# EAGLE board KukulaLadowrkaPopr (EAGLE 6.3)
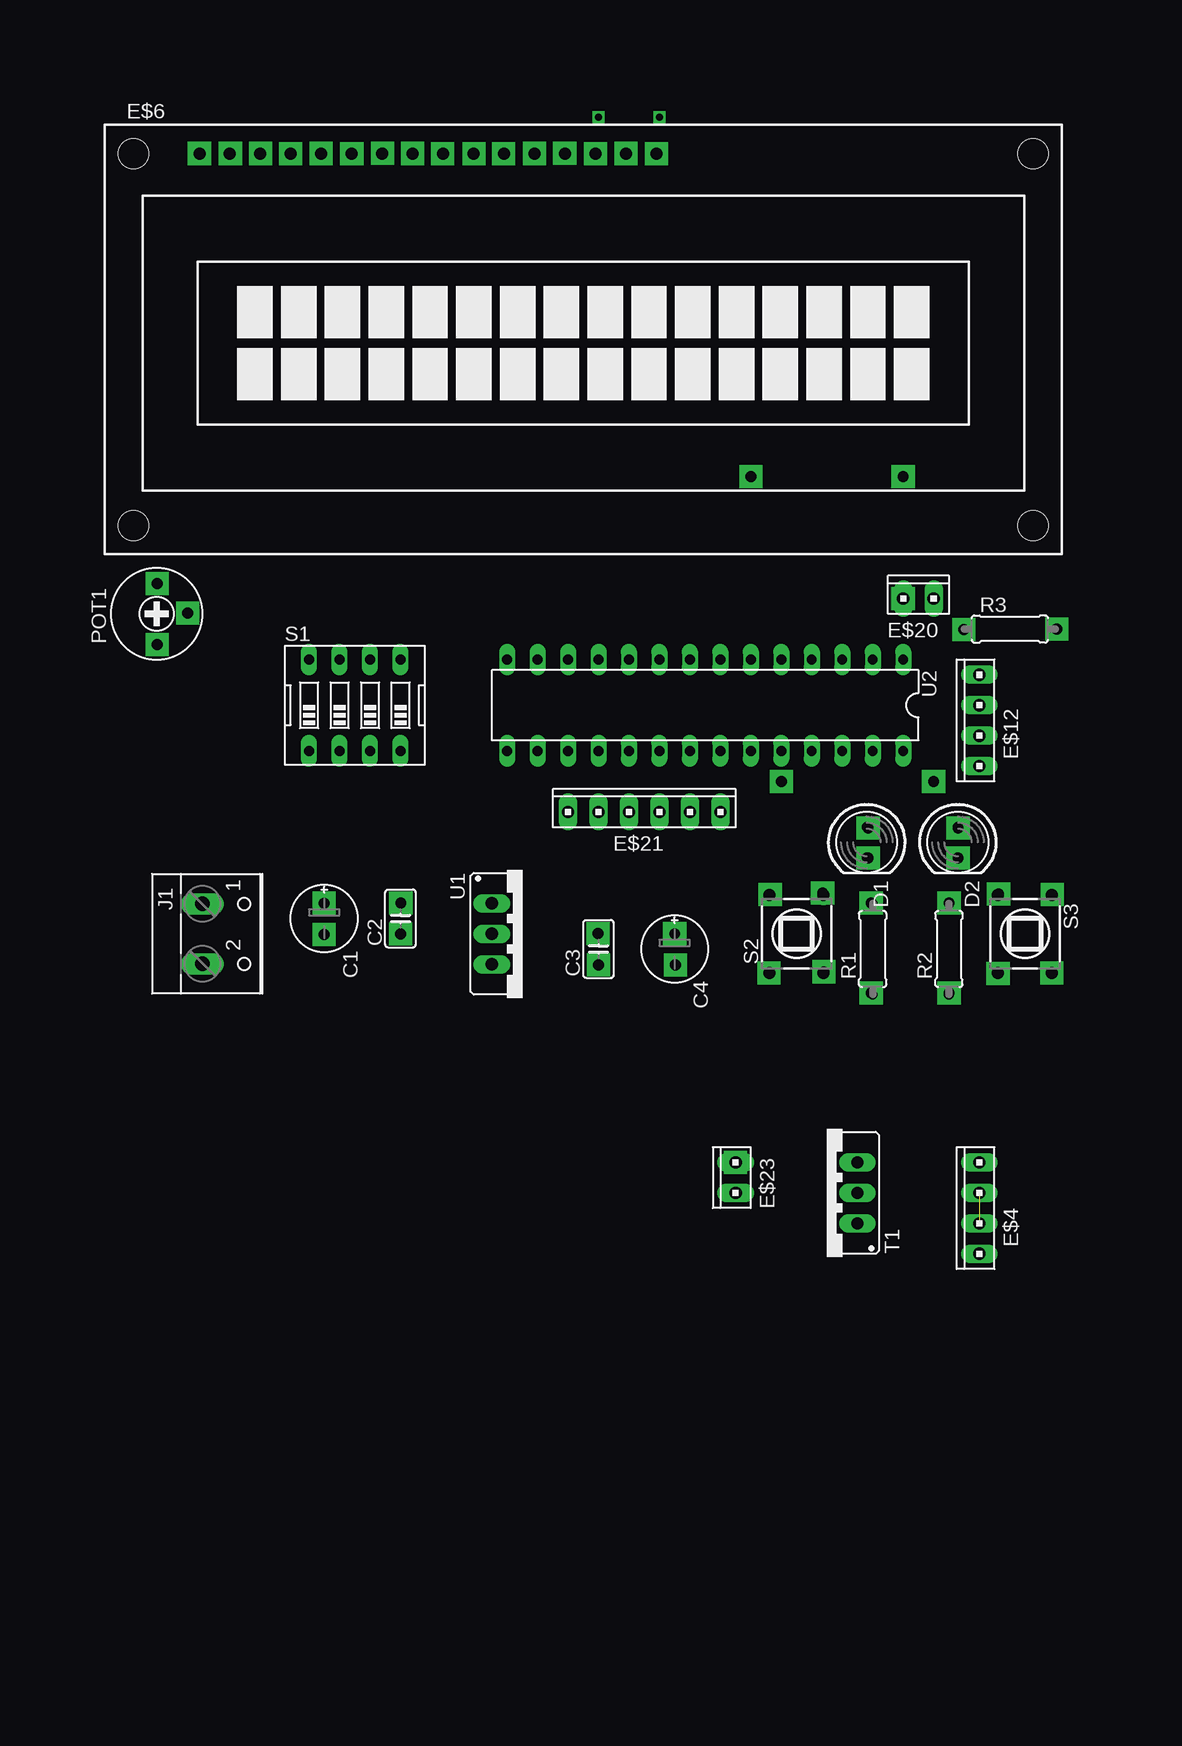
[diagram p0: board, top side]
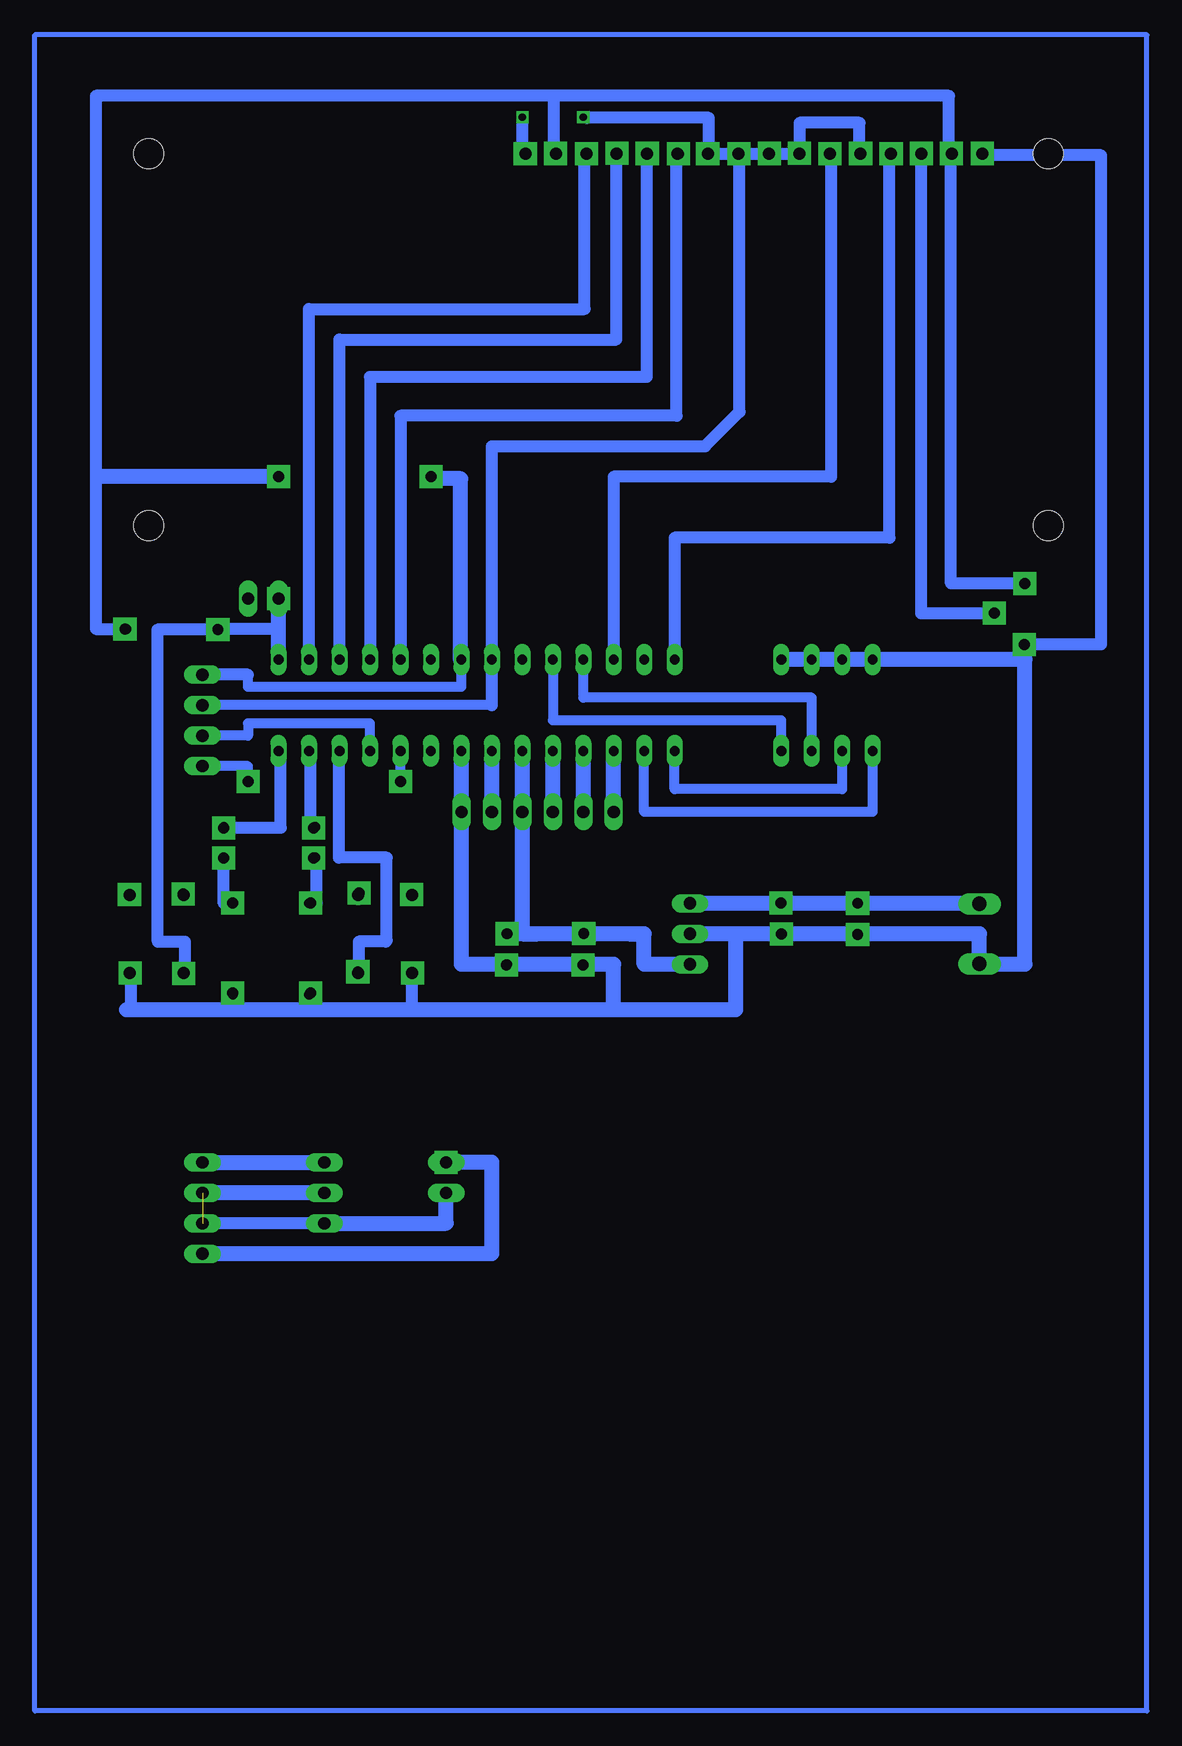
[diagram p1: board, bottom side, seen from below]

No outline drawn. Coordinates in mm, seen from the top.
Copper layers (1*16): Top 0.035mm / dielectric 1.5mm / Bottom 0.035mm
Design rules "default": minimum track width 10mil, minimum drill 24mil, track to track 8mil, track to pad 8mil, pad to pad 8mil, via to via 8mil, smd to smd 8mil, copper to edge 40mil, drill to drill 8mil, minimum pad ring 10mil, minimum via ring 8mil, stop-mask expansion 4mil, vias tented up to drill 0mil, thermal gap 10mil

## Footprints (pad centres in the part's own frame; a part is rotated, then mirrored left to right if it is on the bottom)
E2,5-6E = drill 0.813 pad 1.575: + -1.27,0 | drill 0.813 pad 1.575 octagon: - 1.27,0
C025-025X050 = drill 0.813 octagon: 1 -1.27,0; 2 1.27,0
LED5MM = drill 0.813 octagon: A -1.27,0; K 1.27,0
10X04MTA = drill 1.016 long: 1 3.81,0; 2 1.27,0; 3 -1.27,0; 4 -3.81,0
TUXGR_16X2_R2 = drill 1 pad 1.676: 1 -32,15.5; 2 -29.46,15.5; 3 -26.92,15.5; 4 -24.38,15.5; 5 -21.84,15.5; 6 -19.3,15.5; 7 -16.76,15.5; 8 -14.22,15.5; 9 -11.68,15.5; 10 -9.14,15.5; 11 -6.6,15.5; 12 -4.06,15.5; 13 -1.52,15.5; 14 1.02,15.5; 15 3.56,15.5; 16 6.1,15.5 | hole 2.5: -37.5,-15.5; 37.5,-15.5; -37.5,15.5; 37.5,15.5
10X02MTA = drill 1.016 long: 1 1.27,0; 2 -1.27,0
10X06MTA = drill 1.016 long: 1 6.35,0; 2 3.81,0; 3 1.27,0; 4 -1.27,0; 5 -3.81,0; 6 -6.35,0
W237-102 = drill 1.194 long: 1 -2.5,-1.27; 2 2.5,-1.27
RTRIM3339P = drill 0.61: 1 -2.54,0; 2 0,-2.54; 3 2.54,0
0207/7 = drill 0.813 octagon: 1 -3.81,0; 2 3.81,0
EDG-04 = drill 0.813 long: 1 -3.81,-3.81; 2 -1.27,-3.81; 3 1.27,-3.81; 4 3.81,-3.81; 5 3.81,3.81; 6 1.27,3.81; 7 -1.27,3.81; 8 -3.81,3.81
TL1105SP = drill 1 pad 1.676: 1 -2.25,3.25; 2 2.25,3.25; 3 -2.25,-3.25; 4 2.25,-3.25
78XXS = drill 1.016 long: GND 0,-2.54; IN -2.54,-2.54; OUT 2.54,-2.54
DIL28-3 = drill 0.813 long: 1 -16.51,-3.81; 2 -13.97,-3.81; 3 -11.43,-3.81; 4 -8.89,-3.81; 5 -6.35,-3.81; 6 -3.81,-3.81; 7 -1.27,-3.81; 8 1.27,-3.81; 9 3.81,-3.81; 10 6.35,-3.81; 11 8.89,-3.81; 12 11.43,-3.81; 13 13.97,-3.81; 14 16.51,-3.81; 15 16.51,3.81; 16 13.97,3.81; 17 11.43,3.81; 18 8.89,3.81; 19 6.35,3.81; 20 3.81,3.81; 21 1.27,3.81; 22 -1.27,3.81; 23 -3.81,3.81; 24 -6.35,3.81; 25 -8.89,3.81; 26 -11.43,3.81; 27 -13.97,3.81; 28 -16.51,3.81

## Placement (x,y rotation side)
C1  [E2,5-6E]  10.16,11.43 270 top
C2  [C025-025X050]  16.51,11.43 90 top
C3  [C025-025X050]  33.02,8.89 90 top
C4  [E2,5-6E]  39.37,8.89 270 top
D1  [LED5MM]  55.38,17.78 270 top
D2  [LED5MM]  62.98,17.78 270 top
E$4  [10X04MTA]  64.77,-12.7 90 top
E$6  U3  [TUXGR_16X2_R2]  31.75,59.69 0 top
E$12  [10X04MTA]  64.77,27.94 90 top
E$20  [10X02MTA]  59.69,38.1 0 top
E$21  [10X06MTA]  36.83,20.32 0 top
E$23  [10X02MTA]  44.45,-10.16 90 top
J1  [W237-102]  1.27,10.16 270 top
POT1  [RTRIM3339P]  -3.81,36.83 90 top
R1  [0207/7]  55.88,8.89 90 top
R2  [0207/7]  62.23,8.89 90 top
R3  [0207/7]  67.31,35.56 0 top
S1  [EDG-04]  12.7,29.21 0 top
S2  [TL1105SP]  49.53,10.16 0 top
S3  [TL1105SP]  68.58,10.16 180 top
T1  [78XXS]  52.07,-11.43 90 top
U1  [78XXS]  26.67,10.16 270 top
U2  [DIL28-3]  41.91,29.21 180 top

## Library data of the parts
C1-C4 POT1 R1-R3 = rcl
D1 D2 = led
E$4 E$12 E$20 E$21 E$23 = con-amp
E$6 = display-lcd
J1 = con-wago-500
S1 = special
S2 S3 = switch
T1 U1 = v-reg
U2 = fairchild-semic

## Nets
S$1: POT1.1 S1.5 U1.GND U2.22
S$2: U2.21
S$3: U1.OUT U2.20
S$4: U2.19
S$6: U2.17
S$7: R3.1 U2.1
S$8: U2.4
S$9: U2.5
S$10: U1.IN
S$11: S1.2 U2.15
S$12: S1.1 U2.16
S$13: U2.24
S$14: S1.4
S$15: S1.3
S$16: U2.2
S$17: U2.3
S$19: U2.12
S$21: U2.14
S$24: R3.2
S$26: U2.7
S$69: U2.8
S$72: R1.2
S$73: R2.2
S$87: U2.25
S$88: E$12.4
S$90: E$4.4
S$93: E$4.3 E$23.2 T1.IN
S$94: E$4.1 T1.OUT

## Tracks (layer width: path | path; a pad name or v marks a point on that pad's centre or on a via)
S$1
  Bottom 1.016: -0.24,75.04 -10.16,75.04 -10.16,34.29 POT1.1 -3.81,33.02
  Bottom 1.27: U2.22 43.18,7.62 30.48,7.62 30.48,3.81 27.94,3.81 | 27.94,3.81 20.32,3.81 20.32,10.16 | S1.5 -3.81,33.02 -3.81,7.62 0,7.62 0,10.16 20.32,10.16 | 20.32,10.16 U1.GND | 27.94,3.81 49.53,3.81 | 27.94,3.81 68.58,3.81 | 68.58,3.81 69.85,3.81 | 68.58,3.81 71.12,3.81
S$2
  Bottom 1.27: 40.64,20.32 U2.21
S$3
  Bottom 1.27: 29.21,10.16 28.57,10.16 | 29.21,10.16 38.1,10.16 | 38.1,10.16 36.83,10.16 | 38.1,10.16 U2.20 | U1.OUT 27.94,7.62 27.94,10.16 29.21,10.16
S$4
  Bottom 1.27: 35.56,20.32 U2.19
S$5
  Bottom 1.27: 33.02,20.32 33.02,25.4
S$6
  Bottom 1.27: 30.48,20.32 U2.17
S$7  (via drill 0.9 pad 1.93)
  Bottom 1.016: 58.42,35.56 R3.1
  Bottom 1.27: U2.1 58.42,35.56 v58.42,38.1
S$8
  Bottom 1.016: 27.72,75.13 27.72,56.56 50.8,56.56 U2.4
S$9
  Bottom 1.016: 25.25,75.13 25.25,53.34 48.26,53.34 U2.5
S$10
  Bottom 1.27: 0,12.7 U1.IN
S$11
  Bottom 0.813: U2.15 25.4,22.23 11.43,22.23 S1.2
S$12
  Bottom 0.813: U2.16 27.94,20.32 8.89,20.32 S1.1
S$13  (via drill 0.9 pad 1.93)
  Bottom 0.813: v48.26,22.86 U2.24
S$14
  Bottom 0.813: 35.56,27.94 16.51,27.94 S1.4
S$15
  Bottom 0.813: 33.02,29.84 13.97,29.84 S1.3
S$16
  Bottom 1.016: 32.9,75.21 32.9,62.23 55.88,62.23 U2.2
S$17
  Bottom 1.016: 30.27,75.04 30.27,59.69 53.34,59.69 U2.3
S$18
  Bottom 1.016: 22.61,75.21 22.61,75.16 14.96,75.16
S$19
  Bottom 1.016: 12.34,75.21 12.34,48.26 30.48,48.26 U2.12
S$20
  Bottom 1.016: 10,75.25 10,77.75 15,77.75 15,75.25
S$21
  Bottom 1.016: 7.48,75.21 7.48,43.18 25.4,43.18 U2.14
S$22
  Bottom 1.016: 4.85,75.29 4.85,36.86 -1.32,36.86
S$23
  Bottom 1.016: 2.37,75.04 2.37,39.36 -3.79,39.36
S$24  (via drill 0.9 pad 1.93)
  Bottom 1.016: 2.54,74.93 2.54,80.01 73.66,80.01 73.66,35.56 v71.23,35.56 R3.2
S$25  (via drill 0.9 pad 1.93)
  other vias: 45.72,48.26
S$26
  Bottom 0.813: U2.7 43.18,30.73 60.96,30.73 60.96,31.75
  Bottom 1.016: 60.96,31.75 64.77,31.75
S$27  (via drill 0.9 pad 1.93)
  Bottom 1.016: 55.75,25.25 55.75,18.98 v55.5,18.98
S$28  (via drill 0.9 pad 1.93)
  Bottom 1.27: v39.38,10.16 38,10.16 38,10.28
S$29  (via drill 0.9 pad 1.93)
  other vias: -3.76,34.27
S$30  (via drill 0.9 pad 1.93)
  other vias: -1.24,36.88
S$31  (via drill 0.9 pad 1.93)
  other vias: -3.78,39.34
S$32  (via drill 0.9 pad 1.93)
  other vias: 37.86,75.19
S$33  (via drill 0.9 pad 1.93)
  other vias: 35.32,75.21
S$34  (via drill 0.9 pad 1.93)
  other vias: 32.76,75.19
S$35  (via drill 0.9 pad 1.93)
  other vias: 30.21,75.23
S$36  (via drill 0.9 pad 1.93)
  other vias: 27.69,75.21
S$37  (via drill 0.9 pad 1.93)
  other vias: 25.09,75.17
S$38  (via drill 0.9 pad 1.93)
  other vias: 22.65,75.17
S$39  (via drill 0.9 pad 1.93)
  other vias: 20.03,75.19
S$40  (via drill 0.9 pad 1.93)
  other vias: 17.51,75.21
S$41  (via drill 0.9 pad 1.93)
  other vias: 15.01,75.23
S$42  (via drill 0.9 pad 1.93)
  other vias: 12.46,75.19
S$43  (via drill 0.9 pad 1.93)
  other vias: 9.9,75.21
S$44  (via drill 0.9 pad 1.93)
  other vias: 7.35,75.19
S$45  (via drill 0.9 pad 1.93)
  other vias: 4.84,75.21
S$46  (via drill 0.9 pad 1.93)
  other vias: 2.33,75.21
S$47  (via drill 0.9 pad 1.93)
  other vias: -0.25,75.21
S$48  (via drill 0.9 pad 1.93)
  other vias: 32.98,10.19
S$49  (via drill 0.9 pad 1.93)
  other vias: 33.03,7.55
S$50  (via drill 0.9 pad 1.93)
  other vias: 39.43,7.57
S$51  (via drill 0.9 pad 1.93)
  other vias: 16.54,12.73
S$52  (via drill 0.9 pad 1.93)
  other vias: 16.51,10.14
S$53  (via drill 0.9 pad 1.93)
  other vias: 10.15,12.71
S$54  (via drill 0.9 pad 1.93)
  other vias: 10.15,10.11
S$55
  Bottom 1.016: 70.7,6.79 70.71,3.8 47.29,3.8 | 47.29,3.8 47.28,6.85 | 47.28,3.81 47.29,3.8
S$56
  Bottom 1.016: 68.51,9.64 68.51,35.46
S$57  (via drill 0.9 pad 1.93)
  other vias: 63.48,35.51
S$58
  Bottom 1.016: 53.39,25.36 53.39,16.5 49.4,16.5 49.4,9.61
S$59  (via drill 0.9 pad 1.93)
  other vias: 47.33,13.42
S$60  (via drill 0.9 pad 1.93)
  other vias: 47.24,6.9
S$61  (via drill 0.9 pad 1.93)
  other vias: 51.81,7
S$62  (via drill 0.9 pad 1.93)
  other vias: 51.71,13.57
S$63  (via drill 0.9 pad 1.93)
  other vias: 66.38,13.47
S$64  (via drill 0.9 pad 1.93)
  other vias: 70.85,13.42
S$65  (via drill 0.9 pad 1.93)
  other vias: 66.33,6.85
S$66  (via drill 0.9 pad 1.93)
  other vias: 70.8,6.9
S$67
  Bottom 1.016: 35.47,75.86 35.46,79.76
S$68
  Bottom 1.016: 22.55,75.17 22.55,78.17 32.74,78.17
S$69
  Bottom 0.813: 40.64,29.21 64.77,29.21
  Bottom 1.016: 19.99,75.21 19.99,53.67 22.86,50.8 40.64,50.8 U2.8 40.64,29.21
S$70
  Bottom 1.016: 63.25,35.5 68.54,35.5
S$71  (via drill 0.9 pad 1.93)
  Bottom 1.016: 58.25,25.25 58.25,18.98 v63,18.98
S$72
  Bottom 1.016: 55.25,16.48 55.25,12.7 R1.2
S$73  (via drill 0.9 pad 1.93)
  Bottom 1.016: v63,16.48 63,12.7 R2.2
S$74
  Bottom 1.016: 56,4 56,4.98
S$75
  Bottom 1.016: 62.25,4 62.25,4.98
S$76  (via drill 0.9 pad 1.93)
  other vias: 55.5,16.48
S$77  (via drill 0.9 pad 1.93)
  other vias: 55.75,12.73
S$78  (via drill 0.9 pad 1.93)
  other vias: 62.25,12.73
S$79  (via drill 0.9 pad 1.93)
  other vias: 55.75,5.23
S$80  (via drill 0.9 pad 1.93)
  other vias: 62.25,5.23
S$81
  Bottom 0.406: -13.97,-54.61 -13.97,85.09 78.74,85.09 78.74,-54.61 -13.97,-54.61
S$82
  Bottom 1.016: 16.51,10.22 16.39,10.22
S$83  (via drill 0.9 pad 1.93)
  Bottom 1.27: v58.42,48.26 73.5,48.26
S$84
  Bottom 1.27: 45.75,48.08 43.25,48.08 43.25,32.92
S$85
  Bottom 0.813: 33,30 33,32.75
S$86
  Bottom 0.813: 35.5,28 35.5,33
S$87
  Bottom 0.813: U2.25 50.8,27.69 60.96,27.69 60.96,26.67 64.77,26.67
S$88  (via drill 0.9 pad 1.93)
  Bottom 0.813: E$12.4 60.96,24.13 v60.96,22.86
S$89  (via drill 0.6)
  other vias: 33.02,78.22
S$90  (via drill 0.9 pad 1.93)
  Bottom 1.27: v44.45,-8.89 40.64,-8.89 40.64,-16.51 E$4.4
S$91  (1 unrouted)
  Bottom 1.27: 54.61,-11.43 64.77,-11.43
S$92  (via drill 0.6)
  Bottom 1.016: 38.1,74.93 v38.1,78.22
S$93
  Bottom 1.016: T1.IN E$4.3
  Bottom 1.27: E$23.2 44.45,-13.97 T1.IN
S$94
  Bottom 1.27: E$4.1 T1.OUT
S$95
  Bottom 1.016: 49.5,9.5 51.75,9.5 51.75,7
S$96
  Bottom 1.016: 68.5,9.5 66.25,9.5 66.25,7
